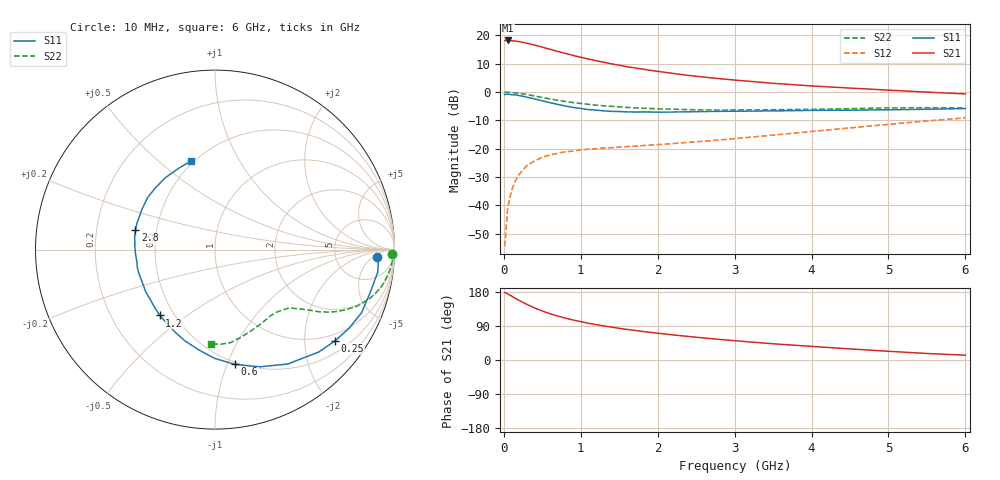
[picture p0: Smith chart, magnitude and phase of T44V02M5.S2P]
! Infineon Technologies  Discrete & RF Semiconductors
! BFR182T
! Si NPN RF Bipolar Junction Transistor in SC75
! VCE = 4 V  IC = 2.5 mA
! Common Emitter S-Parameters:  October  1999
# GHz  S  MA  R  50
!  f  S11  S21  S12  S22
! GHz  MAG  ANG  MAG  ANG  MAG  ANG  MAG  ANG
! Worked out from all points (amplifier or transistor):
!   36 points, 10 MHz to 6 GHz, reference 50 ohm
!   highest |S21| = 18.2 dB at 50 MHz (marker M1)
!   |S21| within 3 dB of that: start of sweep to 585.9 MHz
!   unconditionally stable (mu >= 1): 1.875 GHz to 4.268 GHz
!   at 250 MHz: K = 0.17, MSG = 22.5 dB, |S12| = -27.4 dB
!   at 1.4 GHz: K = 0.84, MSG = 14.8 dB, |S12| = -19.6 dB
!   at 6 GHz: K = 0.83, MSG = 4.2 dB, |S12| = -9.1 dB
!   lowest NFmin = 1.10 dB at 450 MHz
!   S11 on the Smith chart (normalised r, x): 10 MHz: 17, -8; 250 MHz: 0.80, -2.77; 600 MHz: 0.48, -1.07; 1.2 GHz: 0.42, -0.40; 2.8 GHz: 0.38, +0.10; 6 GHz: 0.48, +0.65
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0.01  0.9048 -2.6  8.121 178.1  0.0019 79.1  0.9885 -1.4
0.02  0.9118 -1.8  8.093 178.0  0.0026 86.5  0.9938 -1.2
0.05  0.9155 -7.9  8.14 174.1  0.0091 88.1  0.9911 -3.3
0.1  0.8977 -15.1  8.043 168.7  0.0182 82.6  0.9818 -6.4
0.15  0.8892 -23.3  7.925 162.7  0.0272 77.7  0.9673 -9.5
0.25  0.8403 -37.2  7.516 151.9  0.0427 69.7  0.9276 -15.1
0.3  0.8123 -44.6  7.28 146.8  0.0502 67.5  0.9047 -17.5
0.4  0.7555 -57.5  6.755 137.3  0.0609 60.8  0.8519 -21.7
0.5  0.6993 -69.1  6.207 129.3  0.0705 56.2  0.8024 -24.7
0.6  0.6487 -80.2  5.693 122.1  0.0777 52.5  0.7564 -27.2
0.8  0.566 -99.2  4.818 110.4  0.0882 47.6  0.6814 -30.6
0.9  0.5352 -108.3  4.433 105.5  0.0907 46.2  0.6505 -31.8
1.1  0.4903 -123.4  3.828 96.9  0.0981 44.3  0.6061 -33.6
1.2  0.4787 -130.0  3.568 93.5  0.0997 43.7  0.5858 -34.4
1.4  0.4551 -142.4  3.141 86.7  0.1042 43.7  0.5595 -36.0
1.6  0.4457 -153.8  2.805 80.7  0.1088 44.5  0.5357 -37.4
2.2  0.4438 -177.1  2.13 66.2  0.1232 48.7  0.4982 -43.2
2.8  0.4559 166.4  1.724 54.5  0.1426 53.3  0.4807 -50.4
3.5  0.4645 151.3  1.425 42.8  0.1734 57.4  0.4871 -59.2
4.5  0.478 133.9  1.174 29.3  0.2329 58.9  0.5086 -73.2
5.5  0.4959 114.4  0.998 17.2  0.3087 56.3  0.5284 -86.6
6  0.5115 105.0  0.926 12.7  0.3504 53.3  0.5246 -92.6
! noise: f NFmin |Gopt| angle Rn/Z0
0.45  1.1  0.39  29  0.35
0.9  1.2  0.37  59  0.28
1.8  1.8  0.28  128  0.2
